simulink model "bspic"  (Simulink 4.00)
settings: Solver=ode45  SolverMode=SingleTasking  StartTime=0.0  StopTime=10.0  FixedStep=0.01  RelTol=1e-3

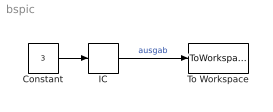
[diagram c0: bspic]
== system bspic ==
  Constant : Constant  Value=3
  IC : InitialCondition  Value=1
  To Workspace : ToWorkspace  VariableName=ausgab  SampleTime=-1  SaveFormat=Array
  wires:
  Constant/1 -> IC/1
  IC/1 -> To Workspace/1  "ausgab"
